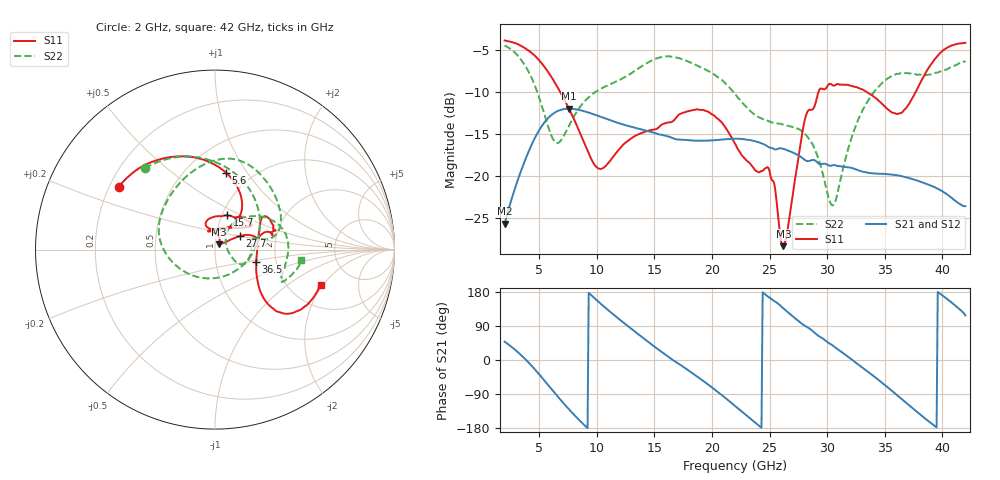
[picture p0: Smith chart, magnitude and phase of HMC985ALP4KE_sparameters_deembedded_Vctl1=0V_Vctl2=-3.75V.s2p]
!s2p File: Measurements: S11, S21, S12, S22
# GHz S dB R 50.0
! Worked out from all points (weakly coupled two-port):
!   401 points, 2 GHz to 42 GHz, reference 50 ohm
!   highest |S21| = -12.01 dB at 7.6 GHz (marker M1); lowest = -25.7 dB at 2 GHz (marker M2)
!   lowest |S11| = -28.4 dB at 26.2 GHz (marker M3), VSWR 1.08, Z = 52.3 + j3.14 ohm
!   |S11| at or under -10 dB: 6.82 GHz to 29.25 GHz (22.43 GHz wide, 124 % of centre); 33.42 GHz to 37.69 GHz (4.271 GHz wide, 12 % of centre)
!   |S22| runs from -23.5 to -4.5 dB; largest |S21 - S12| = 0.00022
!   S11 on the Smith chart (normalised r, x): 2 GHz: 0.24, +0.28; 5.6 GHz: 0.77, +0.81; 15.7 GHz: 1.06, +0.42; 27.7 GHz: 1.30, +0.20; 36.5 GHz: 1.57, -0.23; 42 GHz: 2.95, -1.89
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2  -3.87 147.0  -25.74 48.4  -25.75 48.4  -4.46 130.7
3.6  -4.65 120.2  -18.78 8.0  -18.78 8.0  -6.50 85.5
4.6  -5.66 101.4  -15.58 -23.8  -15.58 -23.8  -9.16 48.8
5.6  -7.28 81.7  -13.40 -59.5  -13.40 -59.5  -13.33 -2.2
6.5  -9.22 66.4  -12.36 -92.4  -12.35 -92.4  -16.09 -69.0
7.6  -12.04 54.6  -12.01 -130.6  -12.01 -130.6  -14.00 -137.4
8.7  -15.41 54.8  -12.23 -165.2  -12.23 -165.2  -11.52 -171.6
10.4  -19.18 89.9  -13.01 146.9  -13.01 146.9  -9.59 161.0
15.4  -14.20 75.7  -15.07 26.7  -15.08 26.7  -5.92 85.8
15.7  -13.87 70.4  -15.14 20.0  -15.14 20.0  -5.82 82.0
19.4  -12.25 33.3  -15.82 -58.7  -15.83 -58.7  -7.31 34.5
22  -16.18 51.3  -15.59 -121.0  -15.59 -121.1  -10.25 11.3
24.9  -19.06 104.5  -16.57 166.5  -16.57 166.5  -13.49 12.7
26.2  -28.41 52.1  -16.80 136.2  -16.80 136.2  -13.91 -3.7
27.7  -16.13 28.6  -17.74 98.1  -17.74 98.1  -14.59 -23.9
28.7  -12.12 12.7  -18.13 77.5  -18.13 77.5  -16.16 -30.6
30.5  -9.22 18.3  -18.74 37.9  -18.75 37.9  -23.54 16.9
32.8  -9.58 33.9  -19.39 -14.3  -19.40 -14.3  -12.98 50.3
35.4  -12.22 11.7  -19.82 -75.8  -19.82 -75.8  -8.29 19.6
36.5  -12.47 -16.7  -20.07 -103.8  -20.07 -103.8  -7.75 6.1
39.5  -5.86 -43.6  -21.49 -178.0  -21.49 -178.0  -7.70 -25.3
42  -4.15 -18.5  -23.64 117.6  -23.65 117.6  -6.32 -6.7
